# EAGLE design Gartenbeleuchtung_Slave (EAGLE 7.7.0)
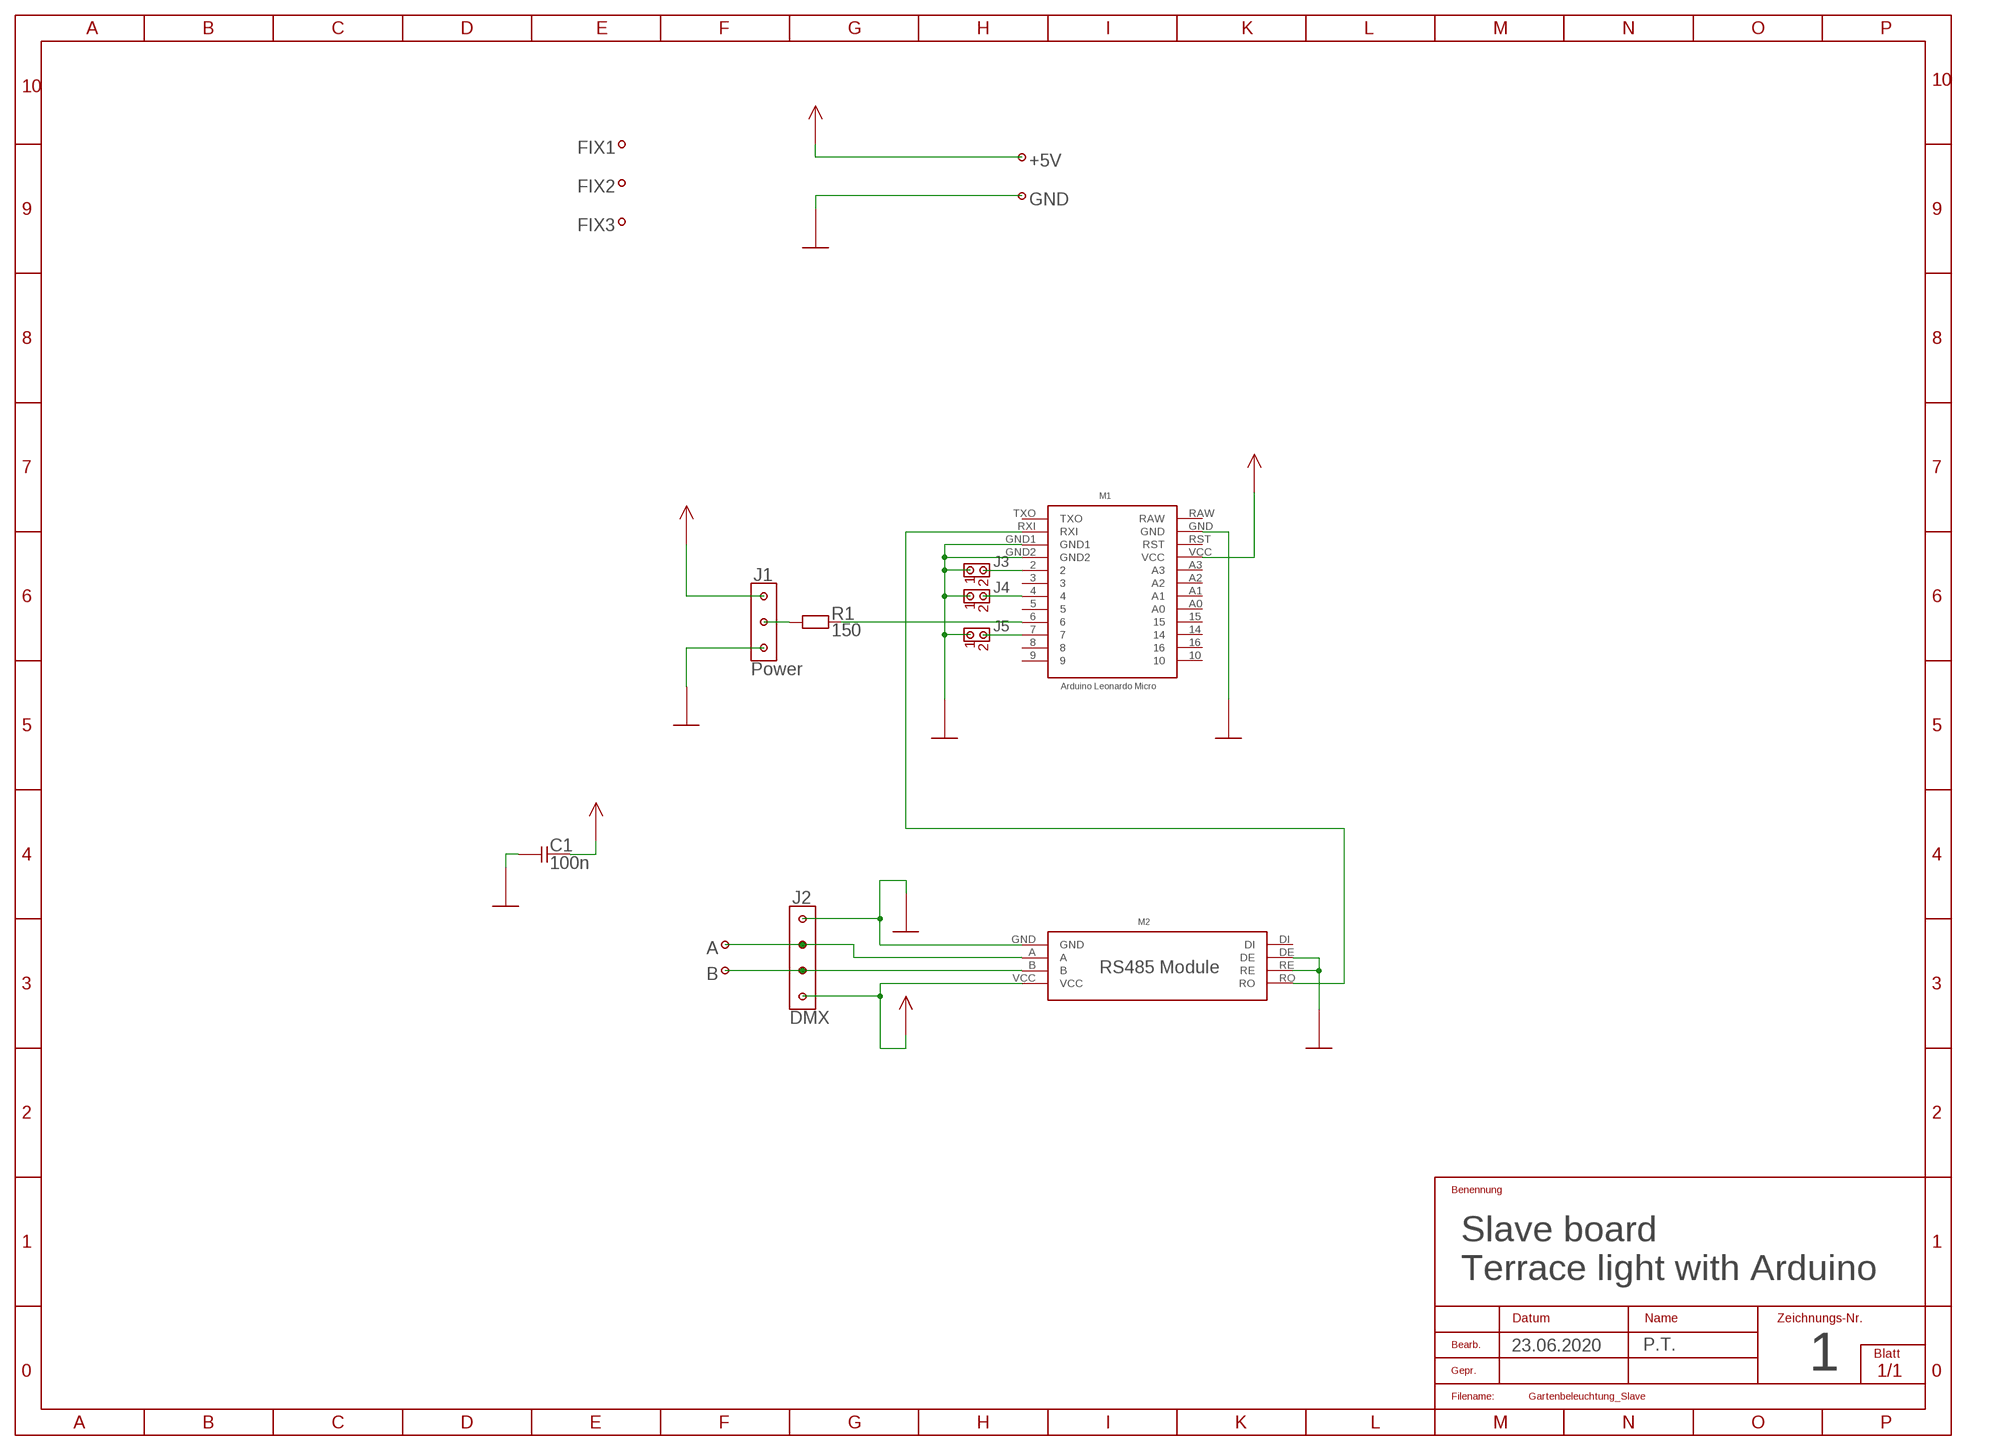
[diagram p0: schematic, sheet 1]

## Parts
+5V  PIN  [PIN]
A  PIN  [PIN]
B  PIN  [PIN]
C1  100n  CAP02  [CAP02B]
FIX1  PIN  [PIN]
FIX2  PIN  [PIN]
FIX3  PIN  [PIN]
GND  PIN  [PIN]
J1  Power  POWER3X1  [POWER3X1]
J2  DMX  POWER4X1  [POWER4X1]
J3  CON02X1  [CON02X1]
J4  CON02X1  [CON02X1]
J5  CON02X1  [CON02X1]
M1  ARDUINO-LEONARDO-MICRO  [ARDUINO-LEONARDO-MICRO]
M2  RS485  [RS485]
R1  150  RES04  [RES04B]

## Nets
GND: C1.1 GND.1 J1.1 J2.4 J3.1 J4.1 J5.1 M1.GND M1.GND1 M1.GND2 M2.DE M2.GND M2.RE
N$1: M1.RXI M2.RO
N$2: M1.6 R1.2
N$3: J1.2 R1.1
N$4: J3.2 M1.2
N$5: A.1 J2.3 M2.A
N$6: B.1 J2.2 M2.B
N$7: J5.2 M1.7
N$8: J4.2 M1.4
VCC: +5V.1 C1.2 J1.3 J2.1 M1.VCC M2.VCC
Unconnected: FIX1.1 FIX2.1 FIX3.1 M1.3 M1.5 M1.8 M1.9 M1.10 M1.14 M1.15 M1.16 M1.A0 M1.A2 M1.A3 M1.RAW M1.RST M1.TXO M2.DI

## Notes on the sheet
- Slave board
- Terrace light with Arduino
- 23.06.2020 | P.T.
- 1

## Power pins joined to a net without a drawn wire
A1: M1.A1

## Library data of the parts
+5V A B FIX1-FIX3 GND = Connector 2:PIN
C1 = Discrete:CAP02
J1 = Connector 2:POWER3X1
J2 = Connector 2:POWER4X1
J3-J5 = Connector 1:CON02X1
M1 = Giess:ARDUINO-LEONARDO-MICRO
M2 = Giess:RS485
R1 = Discrete:RES04

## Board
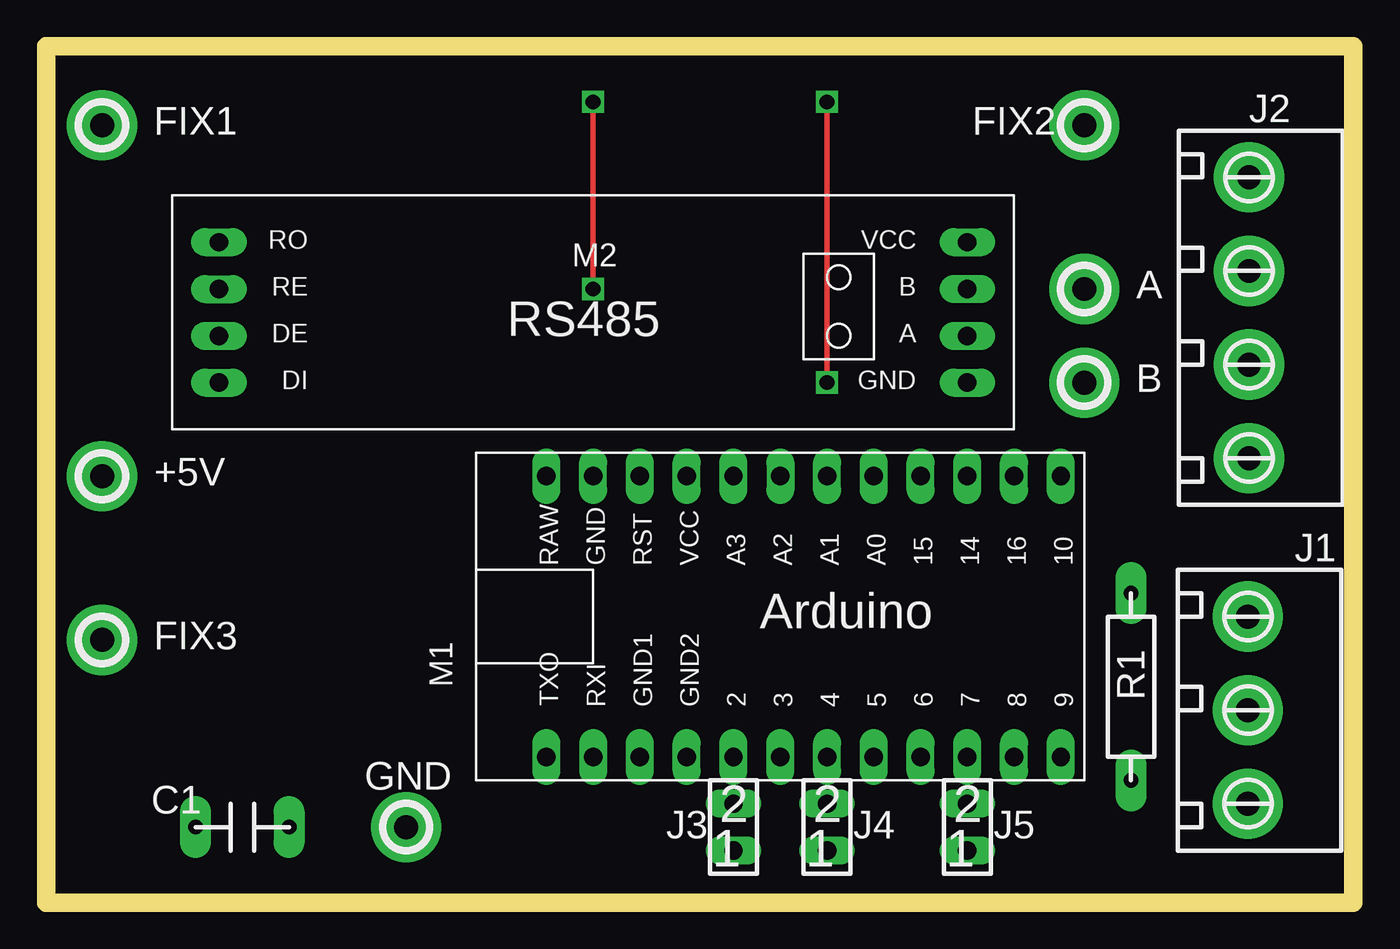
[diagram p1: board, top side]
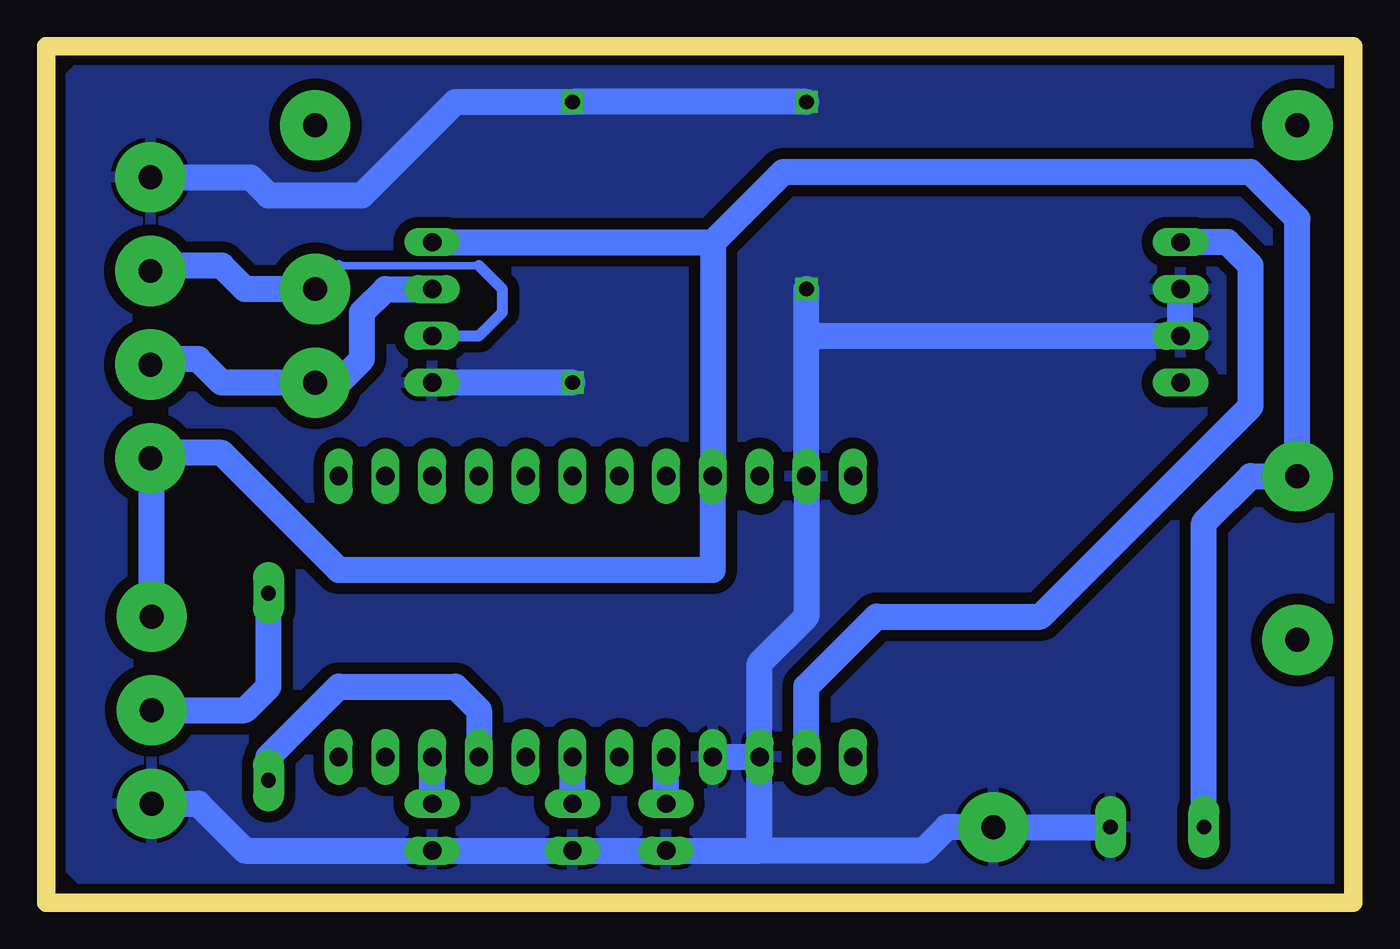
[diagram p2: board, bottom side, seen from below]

Size 71 x 46.5 mm. Coordinates in mm from the lower left corner, seen from the top.
Outline: 0,46.5 71,46.5 71,0 0,0 0,46.5
Copper layers (1*16): Top 0.035mm / dielectric 1.5mm / Bottom 0.035mm
Design rules "default": minimum track width 10mil, minimum drill 24mil, track to track 8mil, track to pad 8mil, pad to pad 8mil, via to via 8mil, smd to smd 8mil, copper to edge 40mil, drill to drill 8mil, minimum pad ring 10mil, minimum via ring 8mil, stop-mask expansion 4mil, vias tented up to drill 0mil, thermal gap 10mil
Milling: 4 lines

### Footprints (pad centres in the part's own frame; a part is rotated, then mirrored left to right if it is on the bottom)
PIN = drill 1.3 pad 3.81: 1 0,0
CAP02B = drill 0.8 pad 1.676 long: 1 0,0; 2 5.08,0
POWER3X1 = drill 1.3 pad 3.81: 1 0,0; 2 0,5.08; 3 0,10.16
POWER4X1 = drill 1.3 pad 3.81: 1 0,0; 2 0,5.08; 3 0,10.16; 4 0,15.24
CON02X1 = drill 1 pad 1.422 long: 1 0,0; 2 0,-2.54
ARDUINO-LEONARDO-MICRO = drill 1 pad 1.422 long: 2 10.16,0; 3 12.7,0; 4 15.24,0; 5 17.78,0; 6 20.32,0; 7 22.86,0; 8 25.4,0; 9 27.94,0; 10 27.94,15.24; 14 22.86,15.24; 15 20.32,15.24; 16 25.4,15.24; A0 17.78,15.24; A1 15.24,15.24; A2 12.7,15.24; A3 10.16,15.24; GND 2.54,15.24; GND1 5.08,0; GND2 7.62,0; RAW 0,15.24; RST 5.08,15.24; RXI 2.54,0; TXO 0,0; VCC 7.62,15.24
RS485 = drill 1 pad 1.422 long: A -20.32,0; B -20.32,-2.54; DE 20.32,0; DI 20.32,2.54; GND -20.32,2.54; RE 20.32,-2.54; RO 20.32,-5.08; VCC -20.32,-5.08
RES04B = drill 0.8 pad 1.676 long: 1 0,0; 2 10.16,0

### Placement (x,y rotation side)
+5V  3.04,23.15 0 top
A  56.38,33.31 0 top
B  56.38,28.23 0 top
C1  13.2,4.1 180 top
FIX1  3.04,42.2 0 top
FIX2  56.38,42.2 0 top
FIX3  3.04,14.26 0 top
GND  19.55,4.1 0 top
J1  65.27,5.37 0 top
J2  65.33,24.13 0 top
J3  37.33,2.83 180 top
J4  42.41,2.83 180 top
J5  50.03,2.83 180 top
M1  27.17,7.91 0 top
M2  29.71,30.77 180 top
R1  58.92,16.8 270 top

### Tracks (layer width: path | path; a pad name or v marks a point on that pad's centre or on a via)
GND  (via drill 0.8 pad 0.61)
  Top 0.305: v42.41,43.47 v42.41,28.23 | v29.71,33.31 v29.71,43.47
  Bottom 1.422: J1.1 62.73,5.37 60.19,2.83 J5.1 J4.1 J3.1 32.25,2.83 | M1.GND2 M1.GND1 | 32.25,2.83 23.36,2.83 22.09,4.1 GND.1 C1.1 | M1.GND1 32.25,12.99 29.71,15.53 M1.GND | M1.GND 29.71,30.77 M2.DE M2.RE | J2.4 59.9,39.37 58.92,38.39 53.84,38.39 48.76,43.47 v42.41,43.47 v29.71,43.47 | v42.41,28.23 M2.GND | M1.GND v29.71,33.31 | 32.25,2.83 M1.GND1
  pour Bottom (isolate 0.61): 1.83,46.01 68.51,46.01 69.84,44.68 69.84,2 68.51,0.67 1.83,0.67 0.5,2 0.5,44.68
N$1
  Bottom 1.422: M1.RXI 29.71,11.72 25.9,15.53 17.01,15.53 5.58,26.96 5.58,34.58 6.85,35.85 M2.RO
N$2
  Bottom 1.422: R1.2 58.92,7.91 55.11,11.72 48.76,11.72 47.49,10.45 M1.6
N$3
  Bottom 1.422: J1.2 60.19,10.45 58.92,11.72 R1.1
N$4
  Bottom 1.422: J3.2 M1.2
N$5
  Bottom 0.406: 47.49,34.58 55.11,34.58
  Bottom 0.61: M2.A 47.49,30.77 46.22,32.04 46.22,33.31 47.49,34.58 | 55.11,34.58 A.1
  Bottom 1.422: A.1 60.19,33.31 61.46,34.58 65.04,34.58 J2.3
N$6
  Bottom 1.422: J2.2 65.04,29.5 62.73,29.5 61.46,28.23 B.1 55.11,28.23 53.84,29.5 53.84,32.04 52.57,33.31 M2.B
N$7
  Bottom 1.422: J5.2 M1.7
N$8
  Bottom 1.422: J4.2 M1.4
VCC
  Bottom 1.422: J1.3 65.27,24.07 J2.1 65.04,24.42 61.46,24.42 55.11,18.07 34.79,18.07 M1.VCC 34.79,35.85 | C1.2 8.12,20.61 5.58,23.15 +5V.1 3.04,37.12 5.58,39.66 30.98,39.66 34.79,35.85 | M2.VCC 34.79,35.85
